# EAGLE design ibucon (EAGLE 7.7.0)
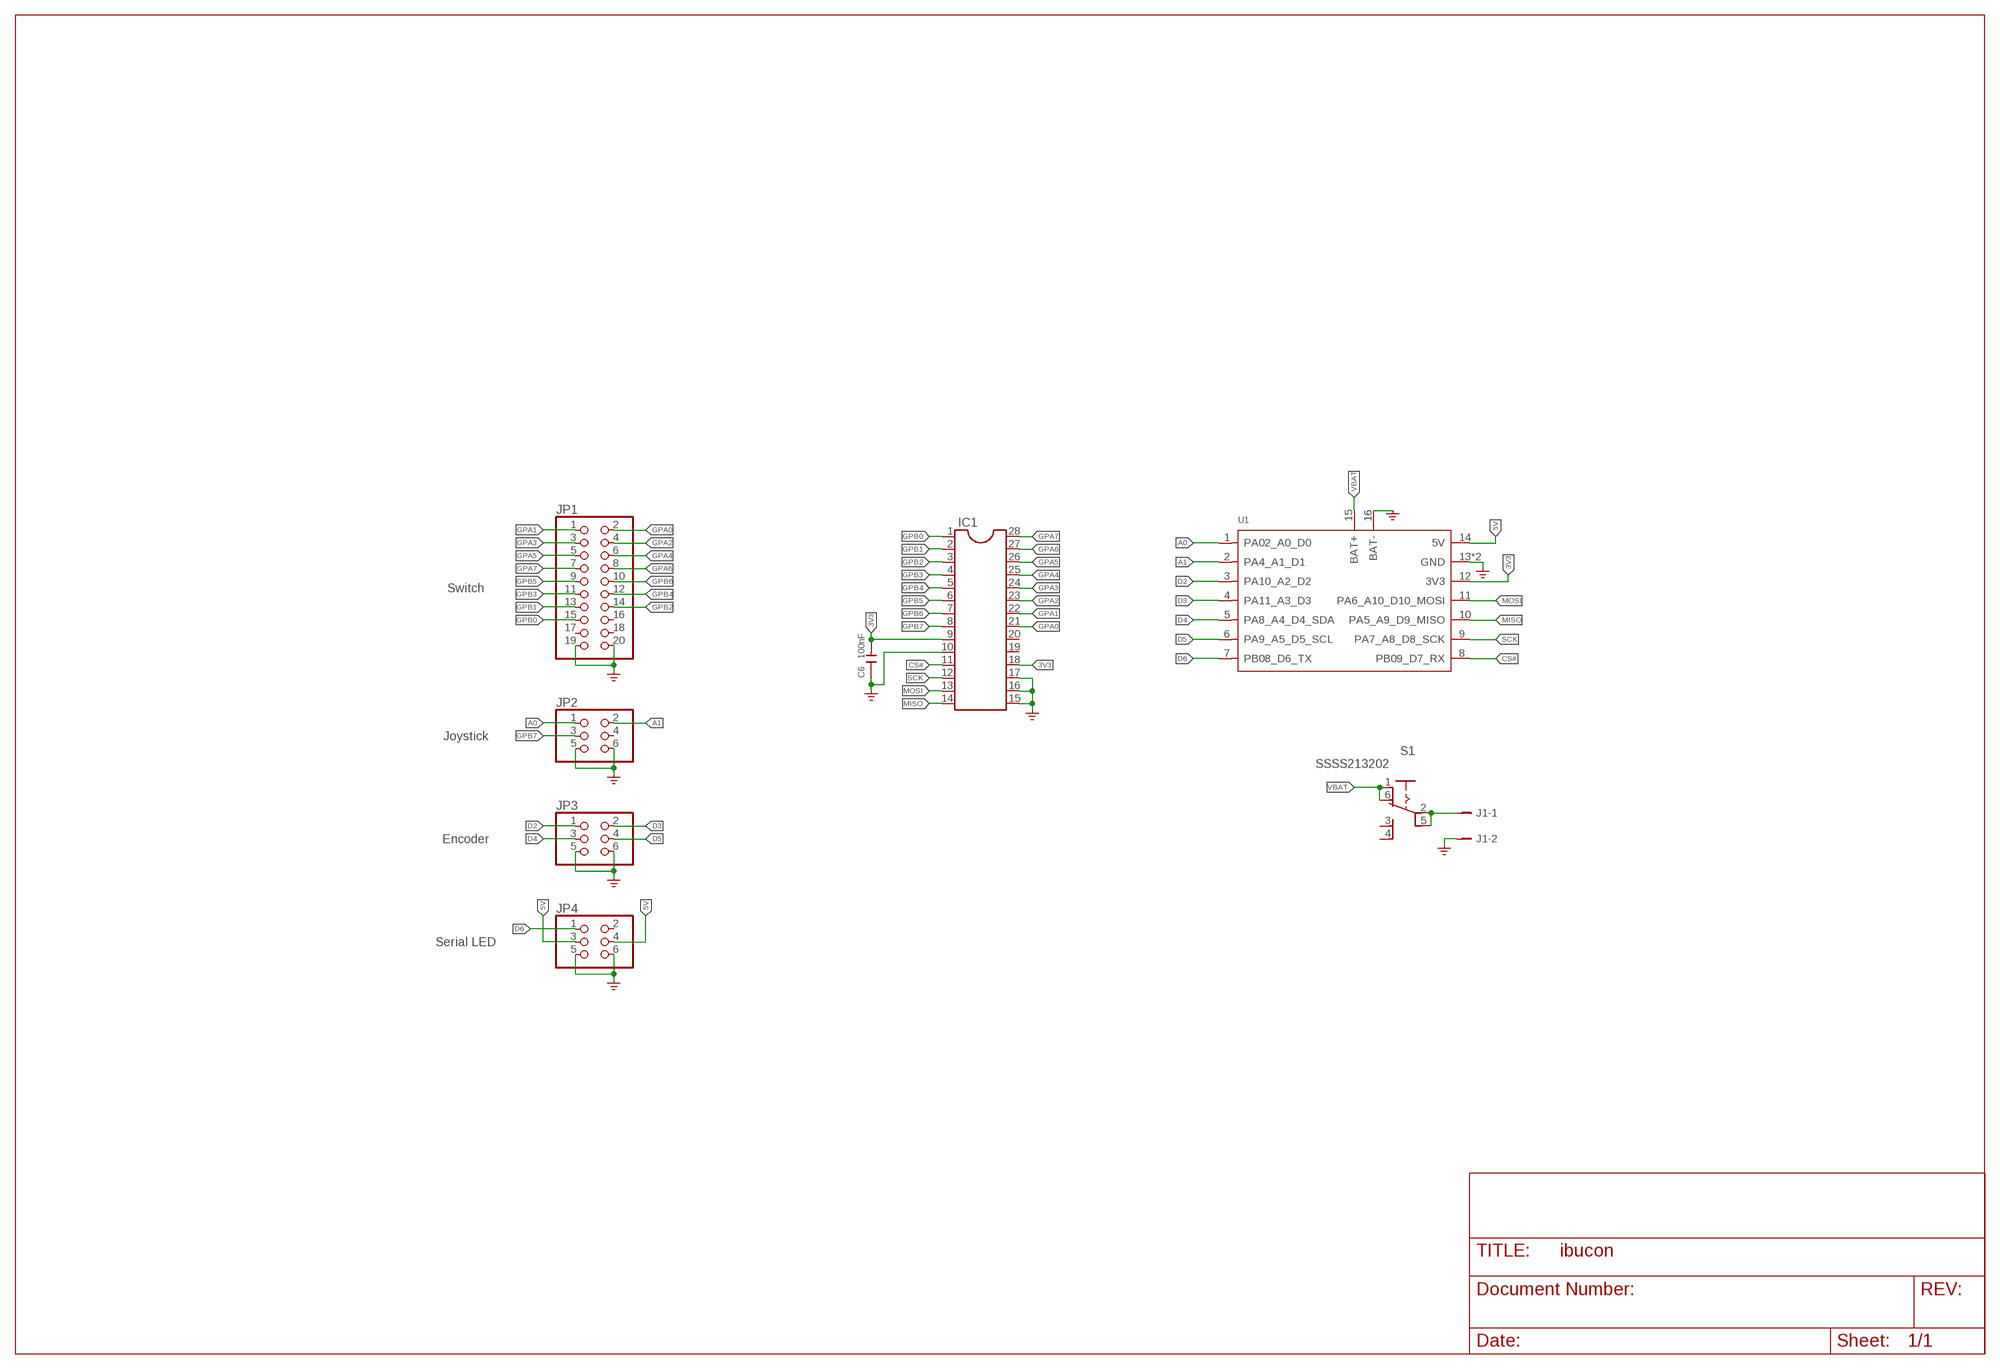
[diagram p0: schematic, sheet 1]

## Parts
C6  100nF  C-0603  [C0603]
IC1  DIL28-3  [DIL28-3]
J1  B2B-PH-K-S  [B2B-PH-K-S]
JP1  PINHD-2X10  [2X10]
JP2  PINHD-2X3  [2X03]
JP3  PINHD-2X3  [2X03]
JP4  PINHD-2X3  [2X03]
S1  SSSS213202  [SSSS213202]
U1  MOUDLE-SEEEDUINO-XIAO-ESP32S3-SMD-TPAD  [MODULE14P-SMD-TPAD]

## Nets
3V3: C6.2 IC1.9 IC1.18 U1.12(3V3)
5V: JP4.3 JP4.4 U1.14(5V)
A0: JP2.1 U1.1(PA02_A0_D0)
A1: JP2.2 U1.2(PA4_A1_D1)
CS#: IC1.11 U1.8(PB09_D7_RX)
D2: JP3.1 U1.3(PA10_A2_D2)
D3: JP3.2 U1.4(PA11_A3_D3)
D4: JP3.3 U1.5(PA8_A4_D4_SDA)
D5: JP3.4 U1.6(PA9_A5_D5_SCL)
D6: JP4.1 U1.7(PB08_D6_TX)
GND: C6.1 IC1.10 IC1.15 IC1.16 IC1.17 J1.2 JP1.19 JP1.20 JP2.5 JP2.6 JP3.5 JP3.6 JP4.5 JP4.6 U1.13(GND) U1.16(BAT-) U1.17(GND) ; supply symbol labelled GND_POWER
GPA0: IC1.21 JP1.2
GPA1: IC1.22 JP1.1
GPA2: IC1.23 JP1.4
GPA3: IC1.24 JP1.3
GPA4: IC1.25 JP1.6
GPA5: IC1.26 JP1.5
GPA6: IC1.27 JP1.8
GPA7: IC1.28 JP1.7
GPB0: IC1.1 JP1.15
GPB1: IC1.2 JP1.13
GPB2: IC1.3 JP1.14
GPB3: IC1.4 JP1.11
GPB4: IC1.5 JP1.12
GPB5: IC1.6 JP1.9
GPB6: IC1.7 JP1.10
GPB7: IC1.8 JP2.3
MISO: IC1.14 U1.10(PA5_A9_D9_MISO)
MOSI: IC1.13 U1.11(PA6_A10_D10_MOSI)
N$1: J1.1 S1.2(C1) S1.5(C2)
SCK: IC1.12 U1.9(PA7_A8_D8_SCK)
VBAT: S1.1(NC1) S1.6(NC2) U1.15(BAT+)
Unconnected: IC1.19 IC1.20 JP1.16 JP1.17 JP1.18 JP2.4 JP4.2 S1.3(NO1) S1.4(NO2)

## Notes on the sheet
- Switch
- Joystick
- Encoder
- Serial LED

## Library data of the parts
C6 = Discrete-small:C*: Ceramic Capacitors
IC1 = ic-package:DIL28: Dual In Line
J1 = con-JST-PH:B2B-PH-K-S: JST-PH 2-way vertical TH; MF: JST; MPN: B2B-PH-K-S
JP1 = pinhead:PINHD-2X10: PIN HEADER
JP2-JP4 = pinhead:PINHD-2X3: PIN HEADER
S1 = matsujirushi:SSSS213202
U1 = Seeed-Studio-XIAO-ESP32S3-footprint-eagle:MOUDLE-SEEEDUINO-XIAO-ESP32S3

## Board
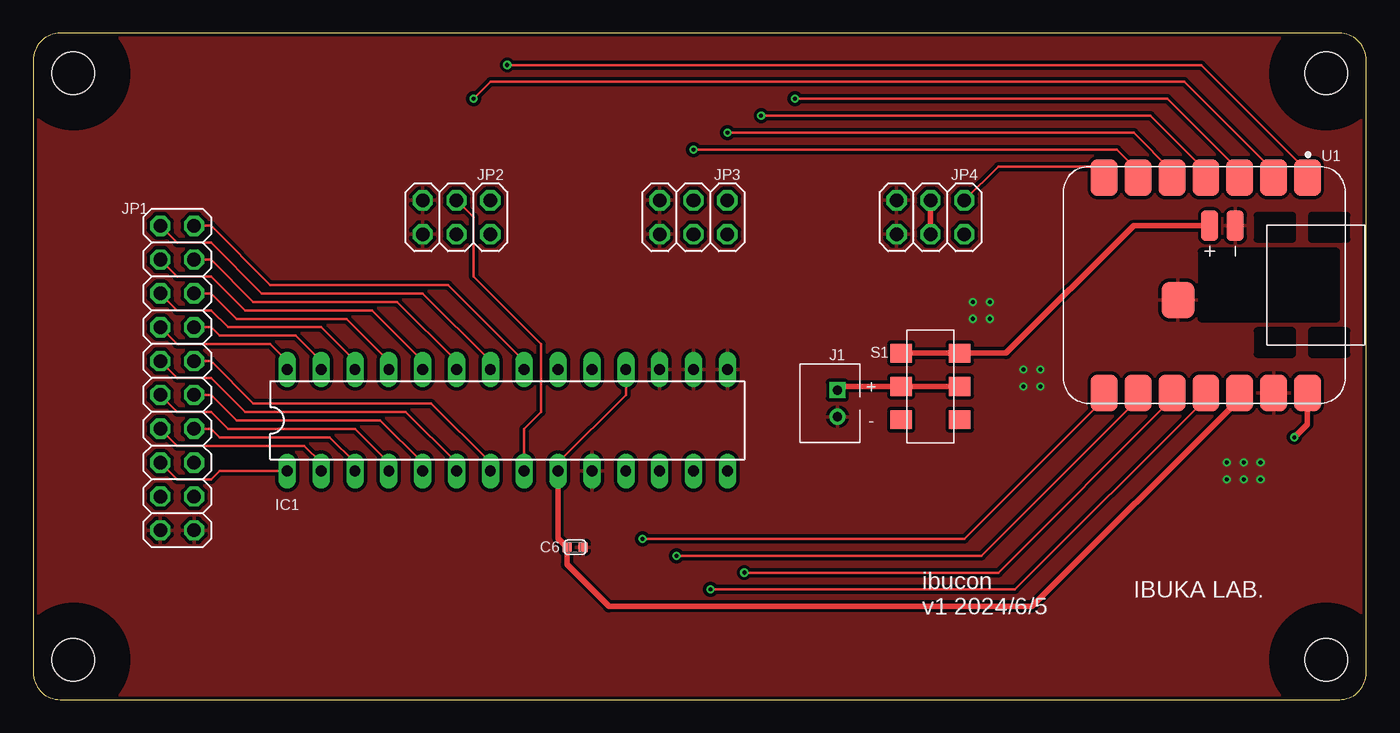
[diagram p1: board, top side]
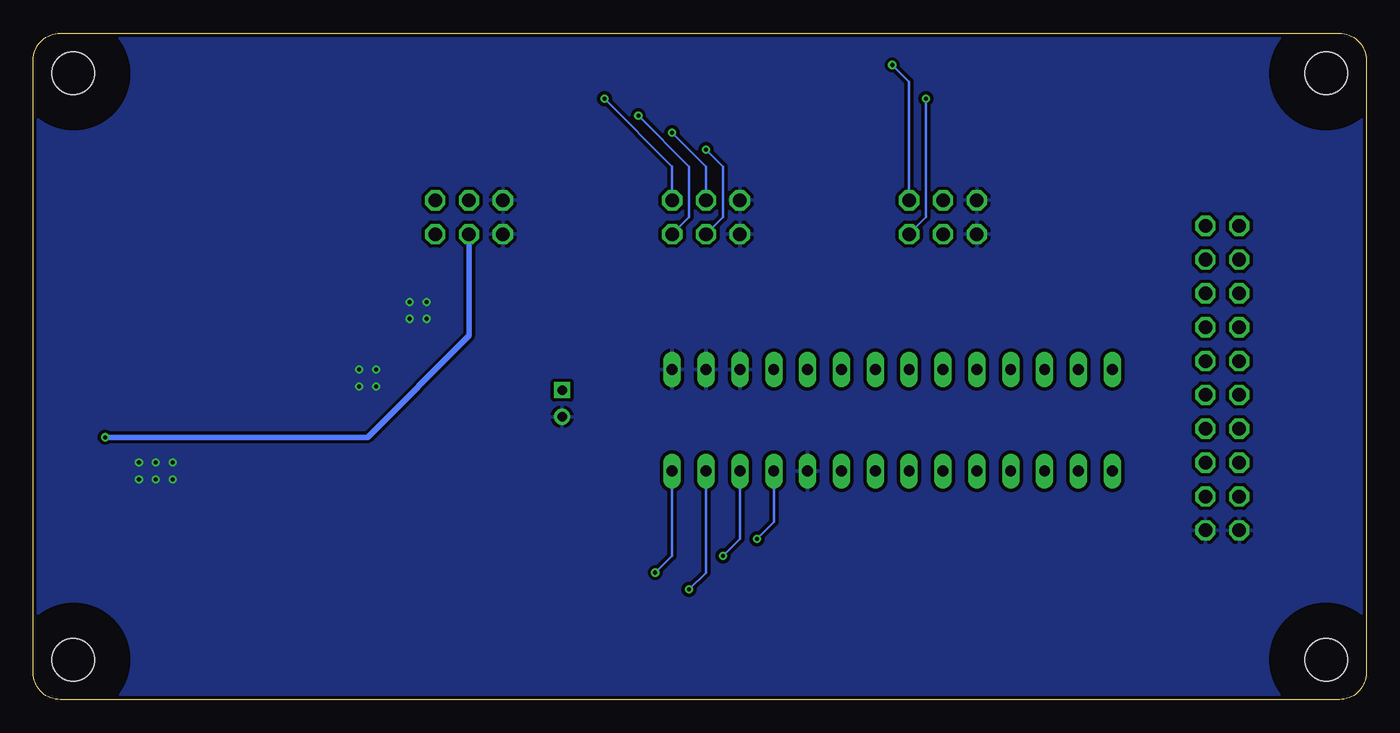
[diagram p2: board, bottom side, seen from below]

Size 100 x 50 mm. Coordinates in mm from the lower left corner, seen from the top.
Outline: 0,48 0,2 arc90 2,0 98,0 arc90 100,2 100,48 arc90 98,50 2,50 arc90 0,48
Copper layers (1*16): Top 0.035mm / dielectric 1.5mm / Bottom 0.035mm
Design rules "SeeedStudio_2layer_DRU_no_angle_20140221": minimum track width 6mil, minimum drill 12mil, track to track 6mil, track to pad 6mil, pad to pad 6mil, via to via 6mil, smd to smd 0mil, copper to edge 10mil, drill to drill 10mil, minimum pad ring 10mil, minimum via ring 6mil, stop-mask expansion 2mil, vias tented up to drill 100mil, thermal gap 10mil
Holes 3.2 mm at 3,3 3,47 97,3 97,47
tRestrict: area -1,-1 to 7,7; area -1,43 to 7,51; area 93,43 to 101,51; area 93,-1 to 101,7
bRestrict: area -1,-1 to 7,7; area -1,43 to 7,51; area 93,43 to 101,51; area 93,-1 to 101,7

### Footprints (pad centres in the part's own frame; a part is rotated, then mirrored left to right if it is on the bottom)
C0603 = smd 0.762 x 0.696: 1 0,0.602; 2 0,-0.602
DIL28-3 = drill 0.813 long: 1 -16.51,-3.81; 2 -13.97,-3.81; 3 -11.43,-3.81; 4 -8.89,-3.81; 5 -6.35,-3.81; 6 -3.81,-3.81; 7 -1.27,-3.81; 8 1.27,-3.81; 9 3.81,-3.81; 10 6.35,-3.81; 11 8.89,-3.81; 12 11.43,-3.81; 13 13.97,-3.81; 14 16.51,-3.81; 15 16.51,3.81; 16 13.97,3.81; 17 11.43,3.81; 18 8.89,3.81; 19 6.35,3.81; 20 3.81,3.81; 21 1.27,3.81; 22 -1.27,3.81; 23 -3.81,3.81; 24 -6.35,3.81; 25 -8.89,3.81; 26 -11.43,3.81; 27 -13.97,3.81; 28 -16.51,3.81
B2B-PH-K-S = drill 0.7 square: 1 1,0 | drill 0.7: 2 -1,0
2X10 = drill 1.016 octagon: 1 -11.43,-1.27; 2 -11.43,1.27; 3 -8.89,-1.27; 4 -8.89,1.27; 5 -6.35,-1.27; 6 -6.35,1.27; 7 -3.81,-1.27; 8 -3.81,1.27; 9 -1.27,-1.27; 10 -1.27,1.27; 11 1.27,-1.27; 12 1.27,1.27; 13 3.81,-1.27; 14 3.81,1.27; 15 6.35,-1.27; 16 6.35,1.27; 17 8.89,-1.27; 18 8.89,1.27; 19 11.43,-1.27; 20 11.43,1.27
2X03 = drill 1.016 octagon: 1 -2.54,-1.27; 2 -2.54,1.27; 3 0,-1.27; 4 0,1.27; 5 2.54,-1.27; 6 2.54,1.27
SSSS213202 = smd 1.4 x 1.6: 1 -2.5,-2.2; 2 0,-2.2; 3 2.5,-2.2; 4 2.5,2.2; 5 0,2.2; 6 -2.5,2.2
MODULE14P-SMD-TPAD = smd 2.75 x 2: 1 0.835,18.12; 2 0.835,15.58; 3 0.835,13.04; 4 0.835,10.5; 5 0.835,7.96; 6 0.835,5.42; 7 0.835,2.88; 8 17,2.88; 9 17,5.42; 10 17,7.96; 11 17,10.5; 12 17,13.04; 13 17,15.58; 14 17,18.12 | smd 2.286 x 1.27: 15 4.445,10.795; 16 4.445,12.7 | smd 2.75 x 2.5: 17 10.01,8.415

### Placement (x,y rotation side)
C6  40.64,11.43 270 top
IC1  35.56,20.95 0 top
J1  60.33,22.23 90 top
JP1  10.79,24.13 270 top
JP2  31.75,36.2 180 top
JP3  49.53,36.2 180 top
JP4  67.31,36.2 180 top
S1  67.31,23.5 270 top
U1  77.47,40.01 270 top

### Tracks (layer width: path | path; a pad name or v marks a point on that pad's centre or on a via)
3V3
  Top 0.203: IC1.9 39.37,17.78 44.45,22.86 IC1.18 | U1.12 90.51,22.57
  Top 0.406: IC1.9 39.37,12.1 C6.2 40.04,10.13 43.18,6.99 74.93,6.99 90.51,22.57
5V  (via drill 0.3)
  Top 0.406: JP4.3 JP4.4 | U1.14 95.59,20.66 v94.61,19.68
  Bottom 0.406: JP4.4 67.31,27.3 74.93,19.68 v94.61,19.68
A0  (via drill 0.3)
  Top 0.203: v35.56,47.62 87.63,47.62 95.59,39.66 U1.1
  Bottom 0.203: JP2.1 34.29,46.35 v35.56,47.62
A1  (via drill 0.3)
  Top 0.203: v33.02,45.09 34.29,46.35 86.36,46.35 93.05,39.66 U1.2
  Bottom 0.203: JP2.2 33.02,36.2 v33.02,45.09
CS#  (via drill 0.3)
  Top 0.203: v45.72,12.06 69.85,12.06 80.35,22.57 U1.8
  Bottom 0.203: v45.72,12.06 44.45,13.34 IC1.11
D2  (via drill 0.3)
  Top 0.203: v57.15,45.09 85.09,45.09 90.51,39.66 U1.3
  Bottom 0.203: JP3.1 52.07,40.01 v57.15,45.09
D3  (via drill 0.3)
  Top 0.203: v54.61,43.81 83.82,43.81 87.97,39.66 U1.4
  Bottom 0.203: JP3.2 50.8,36.2 50.8,40.01 v54.61,43.81
D4  (via drill 0.3)
  Top 0.203: v52.07,42.55 82.55,42.55 85.43,39.66 U1.5
  Bottom 0.203: JP3.3 49.53,40.01 v52.07,42.55
D5  (via drill 0.3)
  Top 0.203: v49.53,41.27 81.28,41.27 82.89,39.66 U1.6
  Bottom 0.203: JP3.4 48.26,36.2 48.26,40.01 v49.53,41.27
D6
  Top 0.203: U1.7 80.35,40.01 72.39,40.01 JP4.1
GND  (via drill 0.3)
  other vias: 92.08,17.78 92.08,16.51 90.81,16.51 90.81,17.78 89.53,17.78 89.53,16.51 75.56,23.5 75.56,24.77 74.3,24.77 74.3,23.5 71.75,28.57 71.75,29.84 70.48,29.84 70.48,28.57
  pour Top (isolate 0.254): 0,50 100,50 100,0 0,0
  pour Bottom (isolate 0.254): 0,50 100,50 100,0 0,0
GPA0
  Top 0.203: JP1.2 13.34,35.56 17.78,31.11 31.11,31.11 36.83,25.4 IC1.21
GPA1
  Top 0.203: JP1.1 10.79,34.29 13.34,34.29 17.14,30.48 29.21,30.48 34.29,25.4 IC1.22
GPA2
  Top 0.203: JP1.4 13.34,33.02 16.51,29.84 27.3,29.84 31.75,25.4 IC1.23
GPA3
  Top 0.203: JP1.3 10.79,31.75 13.34,31.75 15.88,29.21 25.4,29.21 29.21,25.4 IC1.24
GPA4
  Top 0.203: JP1.6 13.34,30.48 15.24,28.57 23.5,28.57 26.67,25.4 IC1.25
GPA5
  Top 0.203: JP1.5 10.79,29.21 13.34,29.21 14.61,27.94 21.59,27.94 24.13,25.4 IC1.26
GPA6
  Top 0.203: JP1.8 13.34,27.94 13.97,27.3 19.68,27.3 21.59,25.4 IC1.27
GPA7
  Top 0.203: JP1.7 10.79,26.67 17.78,26.67 19.05,25.4 IC1.28
GPB0
  Top 0.203: JP1.15 10.79,16.51 13.34,16.51 13.97,17.14 IC1.1
GPB1
  Top 0.203: IC1.2 21.59,17.78 20.32,19.05 10.79,19.05 JP1.13
GPB2
  Top 0.203: IC1.3 24.13,17.78 22.23,19.68 13.97,19.68 13.34,20.32 JP1.14
GPB3
  Top 0.203: JP1.11 10.79,21.59 13.34,21.59 14.61,20.32 24.13,20.32 26.67,17.78 IC1.4
GPB4
  Top 0.203: IC1.5 29.21,17.78 26.04,20.95 15.24,20.95 13.34,22.86 JP1.12
GPB5
  Top 0.203: JP1.9 10.79,24.13 13.34,24.13 15.88,21.59 27.94,21.59 31.75,17.78 IC1.6
GPB6
  Top 0.203: JP1.10 13.34,25.4 16.51,22.23 29.84,22.23 34.29,17.78 IC1.7
GPB7
  Top 0.203: JP2.3 33.02,36.2 33.02,31.75 38.1,26.67 38.1,21.59 36.83,20.32 IC1.8
MISO  (via drill 0.3)
  Top 0.203: v53.34,9.53 72.39,9.53 85.43,22.57 U1.10
  Bottom 0.203: v53.34,9.53 52.07,10.79 IC1.14
MOSI  (via drill 0.3)
  Top 0.203: v50.8,8.26 73.66,8.26 87.97,22.57 U1.11
  Bottom 0.203: v50.8,8.26 49.53,9.53 IC1.13
N$1
  Top 0.406: S1.5 S1.2 60.33,23.5 J1.1
SCK  (via drill 0.3)
  Top 0.203: v48.26,10.79 71.12,10.79 82.89,22.57 U1.9
  Bottom 0.203: v48.26,10.79 46.99,12.06 IC1.12
VBAT
  Top 0.406: S1.1 S1.6 72.98,26 82.55,35.56 U1.15

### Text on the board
tPlace: + | - | ibucon | IBUKA LAB. | v1 2024/6/5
